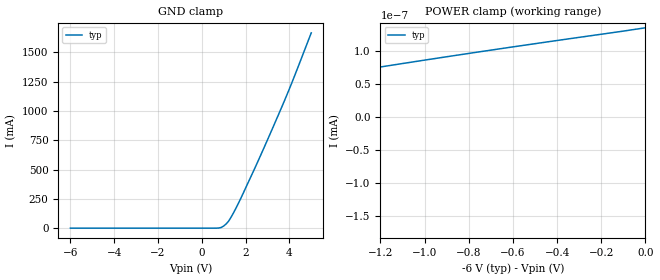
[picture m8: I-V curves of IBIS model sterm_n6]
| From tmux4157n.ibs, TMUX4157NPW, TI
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| sterm_n6
[Model]   sterm_n6
Model_type   Terminator
|   typ   min   max
C_comp   6.976543e-12   NA   NA
[Voltage Range]   -6   NA   NA
[Temperature Range]   27   NA   NA
[Power Clamp Reference]   -6   NA   NA
[GND Clamp Reference]   0   NA   NA
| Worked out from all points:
|   POWER clamp passes 1 mA (typ) near -6.78 V on its own axis
[GND Clamp]
|   Voltage   I(typ)   I(min)   I(max)
-6V       -292.9pA   NA         NA
666.7mV   218.7uA    NA         NA
888.9mV   6.156mA    NA         NA
1V        18.23mA    NA         NA
1.222V    58.7mA     NA         NA
1.444V    128.7mA    NA         NA
1.778V    252.2mA    NA         NA
2.556V    566.3mA    NA         NA
3.889V    1.138A     NA         NA
5V        1.667A     NA         NA
[POWER Clamp]
|   Voltage   I(typ)   I(min)   I(max)
-11V      -1.819A    NA         NA
-4.889V   -180.9pA   NA         NA
-4.778V   -170.8pA   NA         NA
-4.222V   -123pA     NA         NA
-3.556V   -70.87pA   NA         NA
-3.111V   -39.08pA   NA         NA
-2.556V   -2.31pA    NA         NA
-2V       31.53pA    NA         NA
-1.333V   68.78pA    NA         NA
-777.8mV  97.45pA    NA         NA
0V        135.1pA    NA         NA
